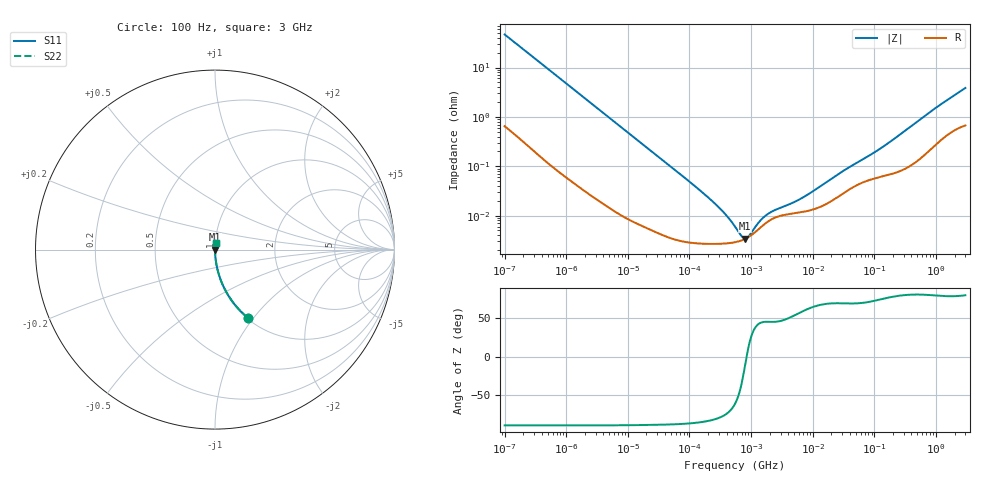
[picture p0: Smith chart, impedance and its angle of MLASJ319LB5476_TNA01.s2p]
! MLASJ319LB5476_TNA01  S-PARAMETER MODEL  ( Standard Model )
! Model Generated by TAIYO YUDEN Corporation (http://www.ty-top.com)
! Version 1.0
! TAIYO YUDEN Control No. 220601
! Copyright(c) 2009 TAIYO YUDEN CO.,LTD. All Rights Reserved.
! Product Description (link to TY-COMPAS)
! https://ds.yuden.co.jp/TYCOMPAS/or/detail?pn=MLASJ319LB5476MTNA01&u=M
! Products Name : Multilayer Ceramic Capacitors
! Characteristics :
!  Capacitance : 47 [uF] , Rated Voltage : 6.3 [V] , TCC : X5R
!  Case Size : 3.2 x 1.6 / 0.126 x 0.063 [mm/inch] , Thickness : 0.85 / 0.033 [mm/inch]
!  (Conditions: Temperature = 25 [degC] , DC Bias Voltage = 0 [V])
! External Node Assignments :
!  1  o---| |---o  2
! GND o---------o GND
! Frequency Range : 100Hz  -  3GHz  [ 401 STEP ]
# MHZ S RI R 50
! Freq[MHz].  S11 Real  S11 Imag  S21 Real  S21 Imag  S12 Real  S12 Imag  S22 Real  S22 Imag
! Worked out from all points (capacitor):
!   401 points, 100 Hz to 3 GHz, reference 50 ohm
!   read as one part in series: C = 33.9 uF near 109 Hz
!   lowest |Z| = 3.44 mohm at 806.9 kHz (marker M1)
!   series resonance near 845 kHz, so ESL is about 1 nH
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0.0001  0.1829 -0.3797  0.8171 0.3797  0.8171 0.3797  0.1829 -0.3797
0.000175  0.0703 -0.2489  0.9297 0.2489  0.9297 0.2489  0.0703 -0.2489
0.000348  0.0197 -0.1328  0.9803 0.1328  0.9803 0.1328  0.0197 -0.1328
0.000724  0.00508 -0.0653  0.9949 0.0653  0.9949 0.0653  0.00508 -0.0653
0.001788  0.00106 -0.0267  0.9989 0.0267  0.9989 0.0267  0.00106 -0.0267
0.031977  4.56e-05 -0.00153  1 0.00153  1 0.00153  4.56e-05 -0.00153
0.16412  2.71e-05 -0.00029  1 0.00029  1 0.00029  2.71e-05 -0.00029
0.2524  2.67e-05 -0.000179  1 0.000179  1 0.000179  2.67e-05 -0.000179
0.388167  2.73e-05 -0.000101  1 0.000101  1 0.000101  2.73e-05 -0.000101
0.441669  2.77e-05 -8.17e-05  1 8.17e-05  1 8.17e-05  2.77e-05 -8.17e-05
0.547723  2.89e-05 -5.26e-05  1 5.26e-05  1 5.26e-05  2.89e-05 -5.26e-05
0.806856  3.4e-05 -5.38e-06  1 5.38e-06  1 5.38e-06  3.4e-05 -5.38e-06
1.53882  6.27e-05 6.27e-05  0.9999 -6.27e-05  0.9999 -6.27e-05  6.27e-05 6.27e-05
1.75092  7.14e-05 7.26e-05  0.9999 -7.26e-05  0.9999 -7.26e-05  7.14e-05 7.26e-05
2.470636  9.16e-05 9.32e-05  0.9999 -9.32e-05  0.9999 -9.32e-05  9.16e-05 9.32e-05
5.361412  0.000113 0.000161  0.9999 -0.000161  0.9999 -0.000161  0.000113 0.000161
9.794414  0.000132 0.000275  0.9999 -0.000275  0.9999 -0.000275  0.000132 0.000275
28.72754  0.000263 0.000706  0.9997 -0.000706  0.9997 -0.000706  0.000263 0.000706
95.87315  0.000559 0.00176  0.9994 -0.00176  0.9994 -0.00176  0.000559 0.00176
175.1444  0.000685 0.00298  0.9993 -0.00298  0.9993 -0.00298  0.000685 0.00298
938.4596  0.00276 0.0142  0.9972 -0.0142  0.9972 -0.0142  0.00276 0.0142
3000  0.00809 0.0375  0.9919 -0.0375  0.9919 -0.0375  0.00809 0.0375
